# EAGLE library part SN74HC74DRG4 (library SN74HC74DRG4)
Dual D-Type Positive-Edge-Triggered Flip-Flops With Clear and Preset Source: Datasheet
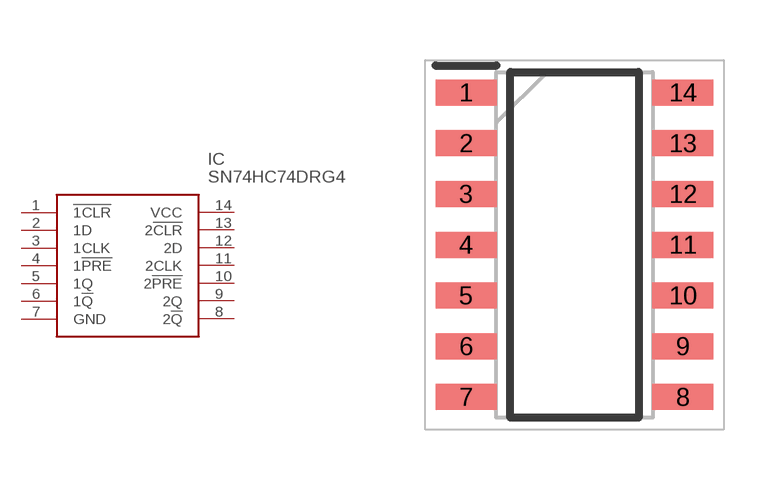
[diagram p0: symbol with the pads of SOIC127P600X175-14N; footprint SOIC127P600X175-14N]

Designator prefix IC

## SN74HC74DRG4 (Description: Dual D-Type Positive-Edge-Triggered Flip-Flops With Clear and Preset; Height: 1.75mm; Manufacturer_Name: Texas Instruments; Manufacturer_Part_Number: SN74HC74DRG4; Mouser_Part_Number: 595-SN74HC74DRG4; Mouser_Price-Stock: https://www.mouser.co.uk/ProductDetail/Texas-Instruments/SN74HC74DRG4?qs=AgY10sKTvDJa4hSfohivVQ%3D%3D)  [SOIC127P600X175-14N]
1  !1CLR
2  1D
3  1CLK
4  1!PRE
5  1Q
6  1!Q
7  GND
8  2!Q
9  2Q
10  2!PRE
11  2CLK
12  2D
13  2!CLR
14  VCC

## Footprint SOIC127P600X175-14N (pad centres in mm)
D (R-PDSO-G14)
smd 1.525 x 0.65: 1 -2.712,3.81; 2 -2.712,2.54; 3 -2.712,1.27; 4 -2.712,0; 5 -2.712,-1.27; 6 -2.712,-2.54; 7 -2.712,-3.81; 8 2.712,-3.81; 9 2.712,-2.54; 10 2.712,-1.27; 11 2.712,0; 12 2.712,1.27; 13 2.712,2.54; 14 2.712,3.81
